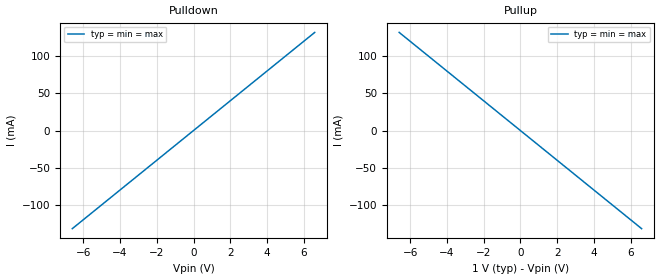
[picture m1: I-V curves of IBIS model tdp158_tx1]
[IBIS Ver]   5.1
[File Name]   tdp158.ibs
[File Rev]   1.0
[Component]   tdp158
[Manufacturer] My Company
[Package]
R_pkg  0.0   NA   NA
L_pkg  0.0   NA   NA
C_pkg  0.0   NA   NA
[Pin]   signal_name   model_name   R_pin L_pin  C_pin
1p   tdp158_tx1_p   tdp158_tx1
1n   tdp158_tx1_n   tdp158_tx1
2p   tdp158_rx1_2p   tdp158_rx1
2n   tdp158_rx1_2n   tdp158_rx1
[Diff_Pin] inv_pin vdiff tdelay_typ tdelay_min tdelay_max
1p   1n   NA   NA   NA   NA
2p   2n   NA   NA   NA   NA
[Model] tdp158_rx1
Model_type Input
C_comp 0p 0p 0p
Vinh = 0.25
Vinl = -0.25
[Temperature_Range] 25 125 0
[Voltage Range] 1.0 1.0 1.0
[Algorithmic Model]
Executable Windows_cl17.00.50727.1_64 tdp158_rx1_x64.dll tdp158_rx1.ami
Executable Windows_cl17.00.50727.1_32 tdp158_rx1.dll tdp158_rx1.ami
[End Algorithmic Model]
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| Models and submodels in the file (2): tdp158_tx1 (Output), tdp158_rx1 (Input)
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[Model] tdp158_tx1
Model_type Output
C_comp 0p 0p 0p
Cref = 0
Vref = 0.5
Rref = 50
Vmeas = 0.5
[Temperature_Range] 25 125 0
[Voltage Range] 1.0 1.0 1.0
[Algorithmic Model]
Executable Windows_cl17.00.50727.1_64 tdp158_tx1_x64.dll tdp158_tx1.ami
Executable Windows_cl17.00.50727.1_32 tdp158_tx1.dll tdp158_tx1.ami
[End Algorithmic Model]
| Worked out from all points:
|   slope of the pulldown table from 0 to 0.15 V, typ, clamps not added: 50 ohm
|   slope of the pullup table from 0 to 0.15 V, typ, clamps not added: 50 ohm
[Pulldown]
-6.6V     -132mA     -132mA     -132mA
0V        0A         0A         0A
6.6V      132mA      132mA      132mA
[Pullup]
-6.6V     132mA      132mA      132mA
0V        0A         0A         0A
6.6V      -132mA     -132mA     -132mA
[GND Clamp]
-6.6V     0A         0A         0A
0V        0A         0A         0A
6.6V      0A         0A         0A
[Power Clamp]
-6.6V     0A         0A         0A
0V        0A         0A         0A
6.6V      0A         0A         0A
[Ramp]
dV/dt_r 0.3/1.5p 0.3/1.5p 0.3/1.5p
dV/dt_f 0.3/1.5p 0.3/1.5p 0.3/1.5p
